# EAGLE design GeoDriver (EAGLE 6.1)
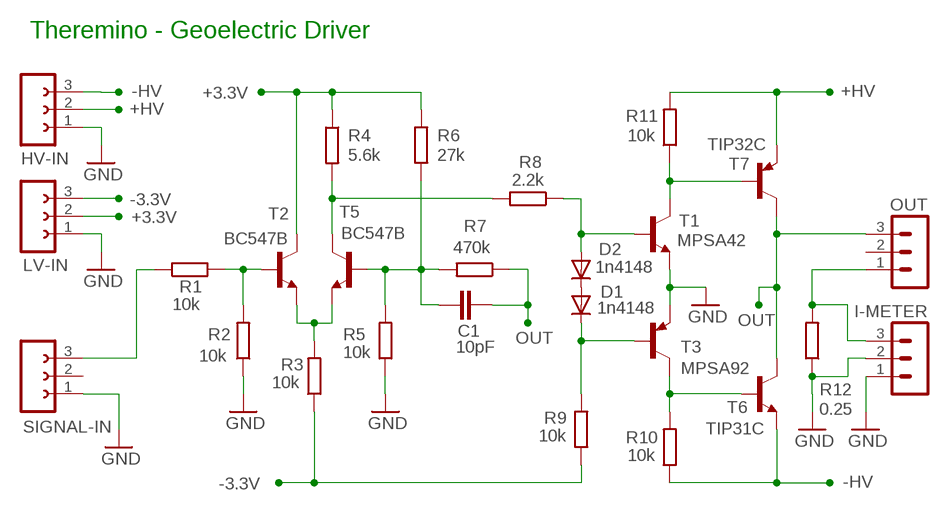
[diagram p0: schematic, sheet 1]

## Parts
C1  10pF  C-EU050-025X075  [C050-025X075]
D1  1n4148  DIODE-D-5  [D-5]
D2  1n4148  DIODE-D-5  [D-5]
HV-IN  FE03-1"  [FE03-1]
I-METER  MA03-1N  [MA03-1]
LV-IN  FE03-1"  [FE03-1]
OUT  MA03-1N  [MA03-1]
R1  10k  R-EU_0204/7  [0204/7]
R2  10k  R-EU_0204/7  [0204/7]
R3  10k  R-EU_0204/7  [0204/7]
R4  5.6k  R-EU_0204/7  [0204/7]
R5  10k  R-EU_0204/7  [0204/7]
R6  27k  R-EU_0204/7  [0204/7]
R7  470k  R-EU_0204/7  [0204/7]
R8  2.2k  R-EU_0204/7  [0204/7]
R9  10k  R-EU_0204/7  [0204/7]
R10  10k  R-EU_0204/7  [0204/7]
R11  10k  R-EU_0204/7  [0204/7]
R12  0.25  R-EU_0207/10  [0207/10]
SIGNAL-IN  FE03-1"  [FE03-1]
T1  MPSA42  -NPN-TO92-EBC  [TO92-EBC]
T2  BC547B  -NPN-TO92-CBE  [TO92-CBE]
T3  MPSA92  -PNP-TO92-EBC  [TO92-EBC]
T5  BC547B  -NPN-TO92-CBE  [TO92-CBE]
T6  TIP31C  -NPN-TO220  [TO220]
T7  TIP32C  -PNP-TO220  [TO220]

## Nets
+3.3V: LV-IN.2 R4.1 R6.2 T2.C
+HV: HV-IN.2 R11.2 T7.3(E)
-3.3V: LV-IN.3 R3.1 R9.1
-HV: HV-IN.3 R10.1 T6.3(E)
GND: HV-IN.1 I-METER.1 I-METER.2 LV-IN.1 R2.1 R5.1 R12.1 SIGNAL-IN.1 T1.E T3.E
N$1: R11.1 T1.C T7.1(B)
N$2: I-METER.3 OUT.1 R12.2
N$3: D1.A D2.C
N$5: D1.C R9.2 T3.B
N$6: R1.1 SIGNAL-IN.3
N$11: R10.2 T3.C T6.1(B)
N$13: R4.2 R8.2 T5.C
N$14: D2.A R8.1 T1.B
N$17: R3.2 T2.E T5.E
N$21: C1.1 R5.2 R6.1 R7.2 T5.B
N$22: R1.2 R2.2 T2.B
OUT: C1.2 OUT.3 R7.1 T6.2(C) T7.2(C)
Unconnected: OUT.2 SIGNAL-IN.2

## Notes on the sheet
- Theremino - Geoelectric Driver

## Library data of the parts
C1 = 00-LIVIO:C-EU: CAPACITOR, European symbol
D1 D2 = 00-LIVIO:DIODE-: DIODE
HV-IN LV-IN SIGNAL-IN = 02-con-lsta-F:FE03-1: FEMALE HEADER
I-METER OUT = 03-con-lstb-M:MA03-1: PIN HEADER
R1-R12 = 00-LIVIO:R-EU_: RESISTOR, European symbol
T1 T2 T5 T6 = 00-LIVIO:*-NPN-: NPN Transistror
T3 T7 = 00-LIVIO:*-PNP-: PNP Transistror

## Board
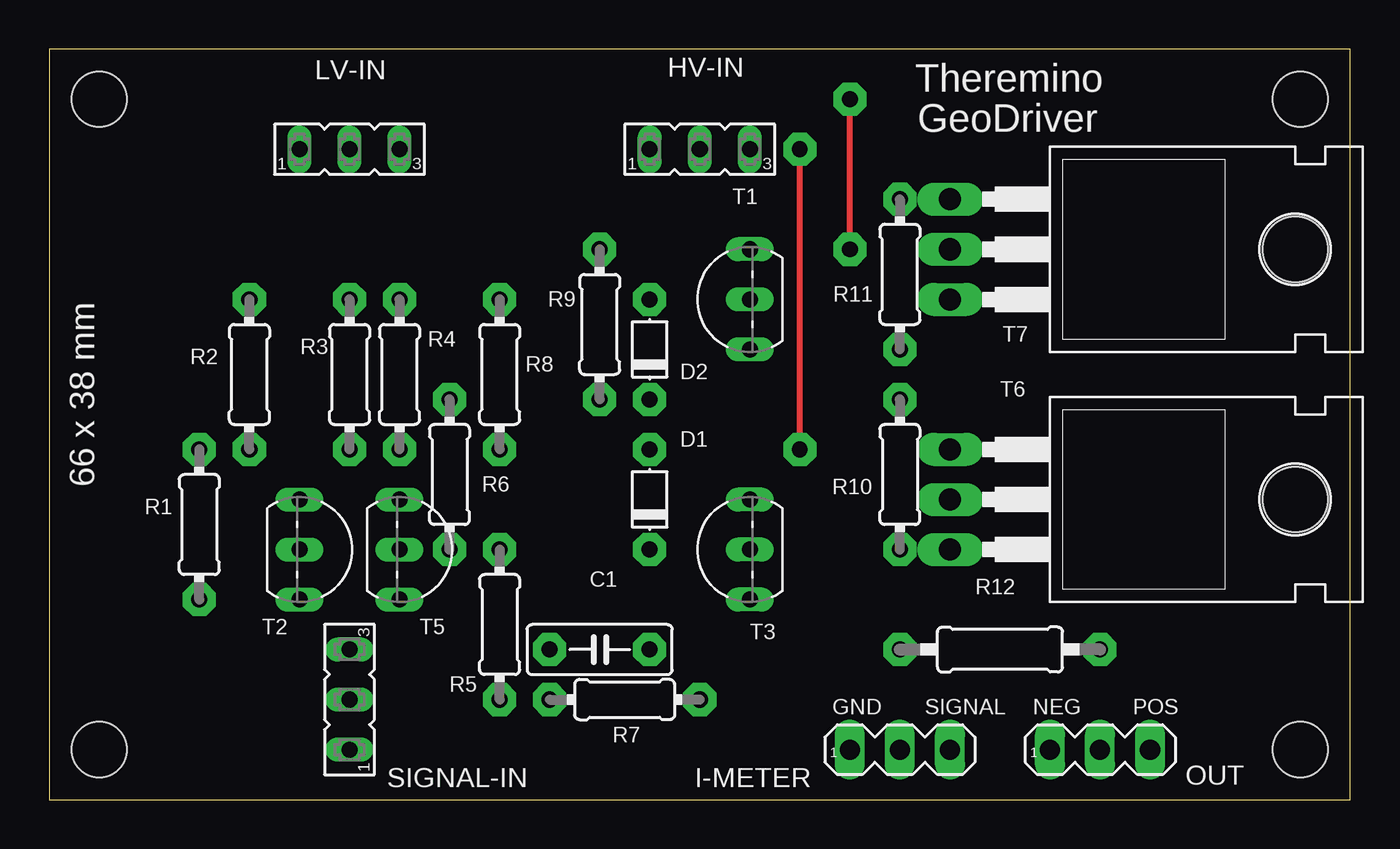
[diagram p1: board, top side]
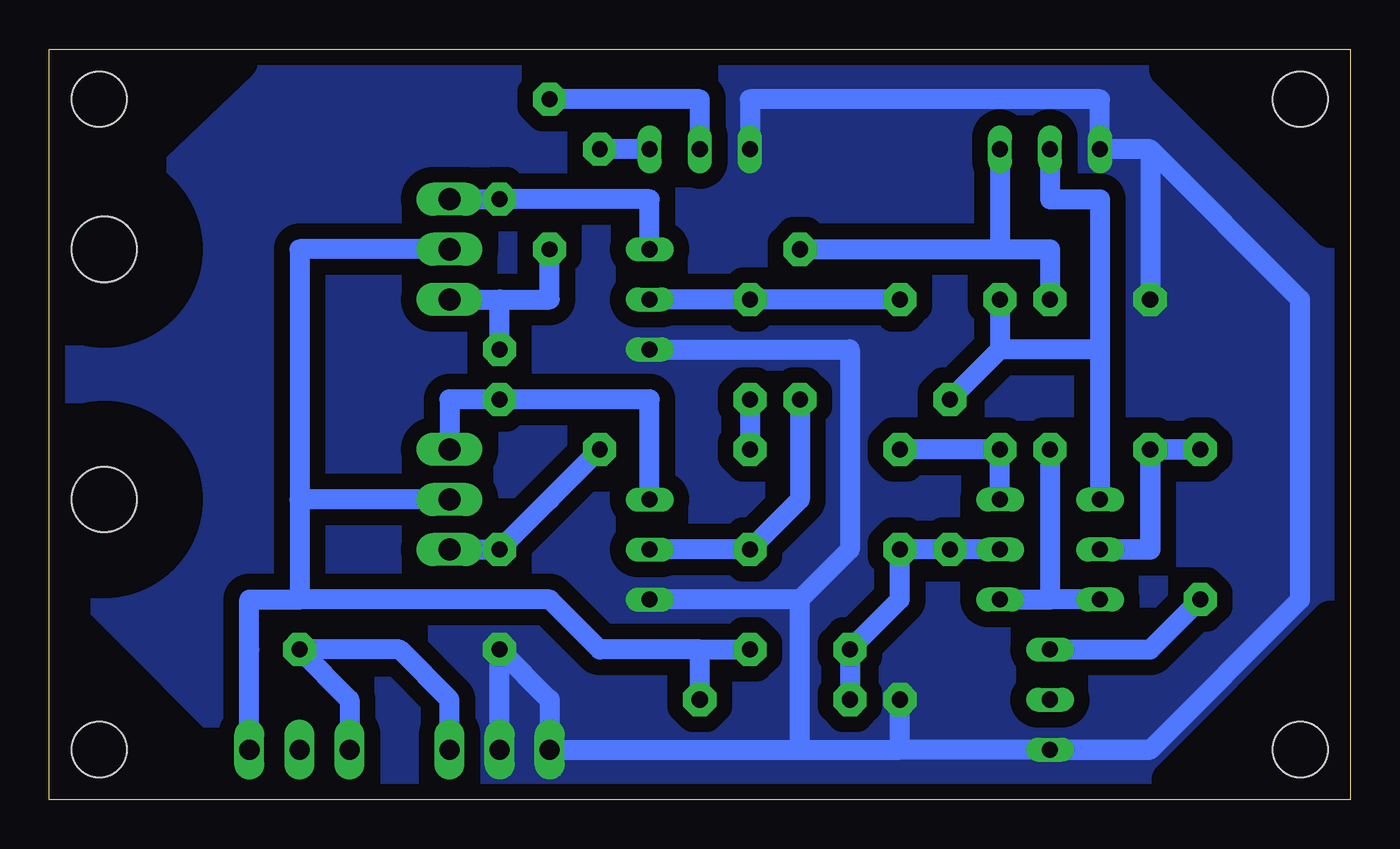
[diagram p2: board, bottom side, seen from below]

Size 66.04 x 38.1 mm. Coordinates in mm from the lower left corner, seen from the top.
Outline: 66.04,38.1 0,38.1 0,0 66.04,0 66.04,38.1
Copper layers (1*16): Top 0.035mm / dielectric 1.5mm / Bottom 0.035mm
Design rules: minimum track width 10mil, minimum drill 0.6mm, track to track 8mil, track to pad 8mil, pad to pad 8mil, via to via 8mil, smd to smd 8mil, copper to edge 31mil, drill to drill 8mil, minimum pad ring 5mil, minimum via ring 8mil, stop-mask expansion 4mil, vias tented up to drill 0mil, thermal gap 41mil
Holes 2.8 mm at 2.54,35.56 2.54,2.54 63.5,2.54 63.5,35.56
bRestrict: 9 lines

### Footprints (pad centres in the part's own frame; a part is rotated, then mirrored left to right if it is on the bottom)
C050-025X075 = drill 0.813 pad 1.676 octagon: 1 -2.54,0; 2 2.54,0
D-5 = drill 0.813 pad 1.676 octagon: A 2.54,0; C -2.54,0
FE03-1 = drill 0.813 long: 1 -2.54,0; 2 0,0; 3 2.54,0
MA03-1 = drill 1.016 long: 1 -2.54,0; 2 0,0; 3 2.54,0
0204/7 = drill 0.813 pad 1.676 octagon: 1 -3.81,0; 2 3.81,0
0207/10 = drill 0.813 pad 1.676 octagon: 1 -5.08,0; 2 5.08,0
TO92-EBC = drill 0.813 long: B 0,0; C 2.54,0; E -2.54,0
TO92-CBE = drill 0.813 long: B 0,0; C -2.54,0; E 2.54,0
TO220 = drill 1.118 long: 1 -2.54,-6.35; 2 0,-6.35; 3 2.54,-6.35 | hole 3.302: 0,11.176

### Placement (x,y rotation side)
C1  27.94,7.62 0 top
D1  30.48,15.24 90 top
D2  30.48,22.86 90 top
HV-IN  33.02,33.02 0 top
I-METER  43.18,2.54 0 top
LV-IN  15.24,33.02 0 top
OUT  53.34,2.54 0 top
R1  7.62,13.97 90 top
R2  10.16,21.59 270 top
R3  15.24,21.59 270 top
R4  17.78,21.59 270 top
R5  22.86,8.89 90 top
R6  20.32,16.51 90 top
R7  29.21,5.08 180 top
R8  22.86,21.59 270 top
R9  27.94,24.13 270 top
R10  43.18,16.51 90 top
R11  43.18,26.67 270 top
R12  48.26,7.62 0 top
SIGNAL-IN  15.24,5.08 90 top
T1  35.56,25.4 90 top
T2  12.7,12.7 270 top
T3  35.56,12.7 90 top
T5  17.78,12.7 270 top
T6  52.07,15.24 270 top
T7  52.07,27.94 270 top

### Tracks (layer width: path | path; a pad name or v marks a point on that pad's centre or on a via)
+3.3V
  Bottom 1.016: 12.7,22.86 17.78,22.86 | LV-IN.2 15.24,30.48 12.7,30.48 12.7,22.86 | 12.7,22.86 17.78,22.86 | 12.7,22.86 T2.C | R6.2 17.78,22.86 | R4.1 17.78,22.86
+HV  (via drill 0.8 pad 1.68)
  Top 0.305: v40.64,27.94 v40.64,35.56
  Bottom 1.016: HV-IN.2 33.02,35.56 v40.64,35.56 | T7.3 43.18,25.4 | 43.18,25.4 40.64,25.4 v40.64,27.94 | R11.2 43.18,25.4
-3.3V
  Bottom 1.016: R9.1 17.78,27.94 | 17.78,27.94 15.24,27.94 R3.1 | LV-IN.3 17.78,27.94
-HV  (via drill 0.8 pad 1.68)
  Top 0.305: v38.1,17.78 v38.1,33.02
  Bottom 1.016: HV-IN.3 v38.1,33.02 | T6.3 R10.1 40.64,15.24 v38.1,17.78
GND
  Bottom 1.016: SIGNAL-IN.1 10.16,2.54 | 10.16,2.54 SIGNAL-IN.1 | SIGNAL-IN.1 22.86,2.54 | 22.86,2.54 R5.1 | 27.94,2.54 22.86,2.54 | T1.E 25.4,22.86 25.4,12.7 27.94,10.16 | 27.94,10.16 T3.E | 27.94,2.54 27.94,10.16 | SIGNAL-IN.1 10.16,2.54 | 10.16,2.54 2.54,10.16 2.54,25.4 10.16,33.02 | 10.16,33.02 LV-IN.1 12.7,35.56 30.48,35.56 HV-IN.1 | 10.16,33.02 R2.1 | 27.94,2.54 I-METER.1 40.64,5.08 R12.1 I-METER.2
  pour Bottom (isolate 0.8, rank 6, no thermals): -1,-1 67.04,-1 67.04,39.1 -1,39.1
N$1
  Bottom 1.016: T7.1 R11.1 35.56,30.48 T1.C
N$2
  Bottom 1.016: OUT.1 50.8,5.08 R12.2 48.26,7.62 45.72,5.08 I-METER.3
N$3
  Bottom 1.016: D2.C D1.A
N$5
  Bottom 1.016: T3.B D1.C 27.94,15.24 R9.2
N$6
  Bottom 1.016: SIGNAL-IN.3 10.16,7.62 R1.1
N$11
  Bottom 1.016: T6.1 45.72,20.32 R10.2 35.56,20.32 T3.C
N$13
  Bottom 1.016: T5.C R4.2 R8.2
N$14
  Bottom 1.016: R8.1 D2.A T1.B
N$17
  Bottom 1.016: R3.2 15.24,16.51 15.24,10.16 | T5.E 15.24,10.16 | T2.E 15.24,10.16
N$21
  Bottom 1.016: T5.B R6.1 | R6.1 R5.2 | R6.1 R5.2 | R7.2 C1.1 22.86,10.16 R5.2
N$22
  Bottom 1.016: R1.2 R2.2 R1.2
  Bottom 1.05: T2.B 10.16,12.7 R2.2
OUT
  Bottom 1.016: R7.1 33.02,7.62 | 33.02,7.62 C1.2 | T7.2 53.34,27.94 53.34,15.24 | 53.34,15.24 53.34,10.16 | T6.2 53.34,15.24 | 33.02,7.62 38.1,7.62 40.64,10.16 53.34,10.16 | OUT.3 55.88,7.62 55.88,10.16 53.34,10.16

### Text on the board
tNames: Theremino | GeoDriver | 66 x 38 mm | GND | SIGNAL | NEG | POS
